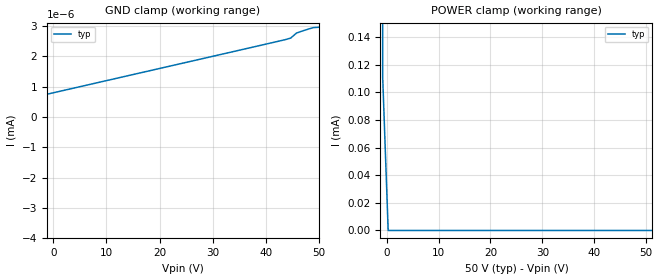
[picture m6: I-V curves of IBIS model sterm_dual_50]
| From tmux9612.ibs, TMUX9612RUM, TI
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| sterm_dual_50
[Model]   sterm_dual_50
Model_type   Terminator
|   typ   min   max
C_comp   6.362683e-12   NA   NA
[Voltage Range]   50   NA   NA
[Temperature Range]   27   NA   NA
[Power Clamp Reference]   50   NA   NA
[GND Clamp Reference]   0   NA   NA
[GND Clamp]
|   Voltage   I(typ)   I(min)   I(max)
-55V      -2.416A    NA         NA
-50.76V   -1.579mA   NA         NA
-49.7V    -1.2nA     NA         NA
43.64V    2.55nA     NA         NA
44.7V     2.605nA    NA         NA
45.76V    2.767nA    NA         NA
48.94V    2.949nA    NA         NA
50V       2.96nA     NA         NA
[POWER Clamp]
|   Voltage   I(typ)   I(min)   I(max)
-5V       1.055A     NA         NA
-1.818V   191.2mA    NA         NA
-757.6mV  111.3uA    NA         NA
303mV     2.957nA    NA         NA
100V      -1.212nA   NA         NA
